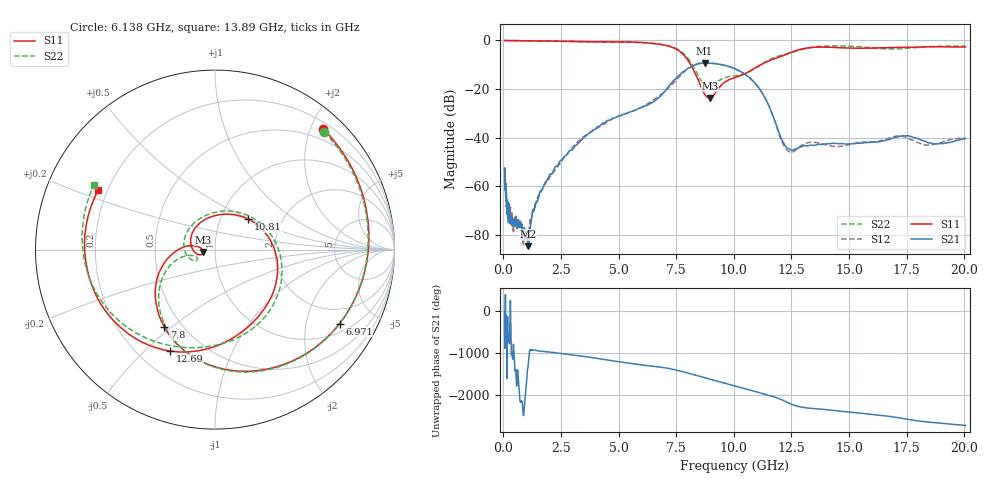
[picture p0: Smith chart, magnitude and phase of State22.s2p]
# Hz S DB R 50
!freq MagS11 AngS11 MagS21 AngS21 MagS12 AngS12 MagS22 AngS22
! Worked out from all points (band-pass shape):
!   1601 points, 50 MHz to 20.05 GHz, reference 50 ohm
!   highest |S21| = -9.22 dB at 8.728 GHz (marker M1); lowest = -84.8 dB at 1.079 GHz (marker M2)
!   |S21| within 3 dB of the highest: 7.915 GHz to 10.18 GHz (2.269 GHz wide, 25.1 % of centre)
!   lowest |S11| = -23.7 dB at 8.96 GHz (marker M3), VSWR 1.14, Z = 44 - j1.23 ohm
!   |S11| at or under -10 dB: 8.129 GHz to 11.16 GHz (3.035 GHz wide, 31.5 % of centre)
!   |S22| runs from -19.2 to 0.0 dB; largest |S21 - S12| = 0.022
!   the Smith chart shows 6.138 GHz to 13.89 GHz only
!   S11 on the Smith chart (normalised r, x): 6.138 GHz: 0.30, +2.19; 6.971 GHz: 1.32, -3.12; 7.8 GHz: 0.40, -0.47; 10.81 GHz: 1.36, +0.49; 12.69 GHz: 0.33, -0.60; 13.89 GHz: 0.16, +0.24
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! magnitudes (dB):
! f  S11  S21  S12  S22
! 50 MHz  0.0  -53.0  -54.3  0.0
! 135.9 MHz  0.0  -68.0  -66.2  0.0
! 194.1 MHz  0.0  -68.1  -73.3  0.0
! 209.2 MHz  0.0  -73.8  -72.3  0.0
! 244.8 MHz  0.0  -67.8  -71.4  0.0
! 369.6 MHz  0.0  -74.3  -71.8  0.0
! 429.4 MHz  0.0  -75.2  -77.3  0.0
! 491.4 MHz  -0.1  -74.8  -73.2  -0.1
! 1.005 GHz  -0.1  -81.5  -79.3  -0.1
! 1.079 GHz  -0.1  -84.8  -79.5  -0.1
! 2.722 GHz  -0.3  -47.4  -47.1  -0.4
! 6.138 GHz  -0.9  -27.0  -26.7  -1.0
! 6.971 GHz  -1.9  -21.3  -21.2  -1.9
! 7.402 GHz  -3.1  -16.4  -17.2  -3.0
! 7.8 GHz  -5.8  -12.8  -13.4  -5.3
! 8.728 GHz  -22.1  -9.2  -9.2  -18.5
! 8.96 GHz  -23.7  -9.3  -9.2  -19.1
! 10.81 GHz  -12.0  -16.4  -16.4  -12.2
! 12.23 GHz  -5.9  -43.4  -44.2  -5.6
! 12.69 GHz  -4.2  -44.7  -45.0  -4.4
! 13.89 GHz  -2.7  -42.8  -42.7  -2.3
! 20.05 GHz  -2.7  -40.5  -40.2  -2.3
